TYPE ST_SlaveStateInfoScanned :
STRUCT
	nIndex 			: DINT;
	sName 			: STRING; 		(* name of slave given in System Manager *)
	sType 			: STRING;		(* type of slave, e.g. EK1100*)
	nECAddr 		: UINT;			(* EtherCAT Slave Addr *)
	bDifferentName	: BOOL;			(* Name of Scanned configuration differs from Configured configuration *)
	bDifferentType	: BOOL;			(* Type Of Scanned configuration differs from Configured configuration *)
	bDifferentAddr	: BOOL;			(* EcAddress of Scanned configuration differs from Configured configuration *)
END_STRUCT
END_TYPE
